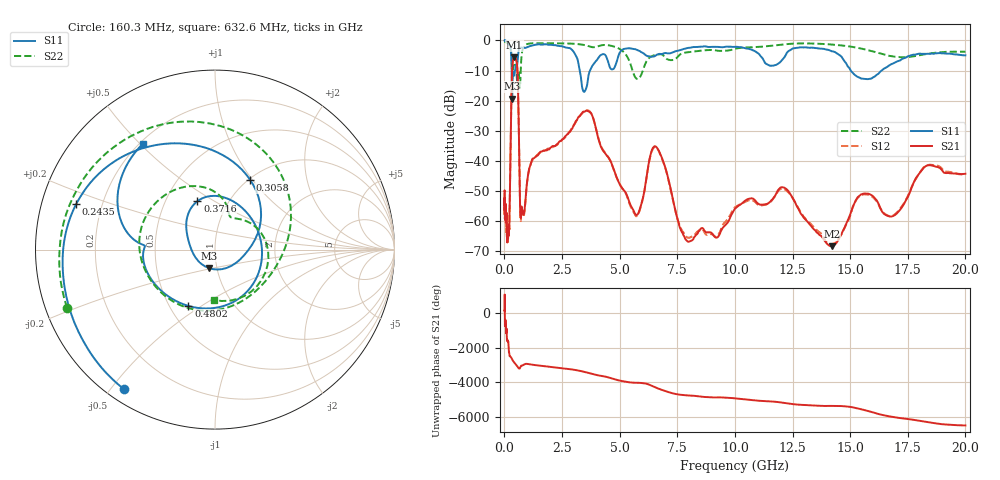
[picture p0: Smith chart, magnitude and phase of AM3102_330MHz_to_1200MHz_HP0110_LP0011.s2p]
! Date/Time: Tue, Sep 11, 2018 5:14 PM
! Network Analyzer: Agilent Technologies E8362B Rev: A.07.50.63
! Sweep from 0.010 to 20.000 GHz, 1601 Points, Sweep Type: LOG
! Power Supply: 4.949 V, 0.001 A
# Hz S DB R 50
!freq MagS11 AngS11 MagS21 AngS21 MagS12 AngS12 MagS22 AngS22
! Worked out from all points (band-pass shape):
!   1601 points, 10 MHz to 20 GHz, reference 50 ohm
!   highest |S21| = -5.58 dB at 426.5 MHz (marker M1); lowest = -68.3 dB at 14.21 GHz (marker M2)
!   |S21| within 3 dB of the highest: 343.4 MHz to 555.1 MHz (211.7 MHz wide, 47.1 % of centre)
!   lowest |S11| = -19.3 dB at 337.9 MHz (marker M3), VSWR 1.24, Z = 45.7 - j9.53 ohm
!   |S11| at or under -10 dB: 315 MHz to 461.3 MHz (146.3 MHz wide, 37.7 % of centre); 3.274 GHz to 3.714 GHz (440.5 MHz wide, 12.6 % of centre); 15.03 GHz to 16.37 GHz (1.34 GHz wide, 8.54 % of centre)
!   |S22| runs from -15.8 to -0.2 dB; largest |S21 - S12| = 0.0081
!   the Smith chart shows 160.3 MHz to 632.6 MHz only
!   S11 on the Smith chart (normalised r, x): 160.3 MHz: 0.05, -0.54; 243.5 MHz: 0.11, +0.16; 305.8 MHz: 1.02, +0.97; 371.6 MHz: 0.72, +0.42; 480.2 MHz: 0.62, -0.44; 632.6 MHz: 0.21, +0.51
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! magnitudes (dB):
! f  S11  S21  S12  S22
! 10 MHz  0.0  -50.1  -50.7  -0.2
! 35.55 MHz  0.0  -57.7  -56.3  -0.4
! 126.4 MHz  -0.4  -65.0  -62.6  -0.9
! 160.3 MHz  -0.6  -65.8  -64.9  -1.1
! 243.5 MHz  -1.8  -48.7  -48.7  -1.9
! 305.8 MHz  -7.2  -18.7  -18.7  -4.6
! 337.9 MHz  -19.3  -9.4  -9.4  -8.6
! 371.6 MHz  -10.8  -6.6  -6.7  -9.6
! 426.5 MHz  -11.6  -5.6  -5.6  -7.8
! 447.2 MHz  -10.7  -5.6  -5.7  -7.4
! 480.2 MHz  -9.2  -5.8  -5.9  -7.6
! 567.1 MHz  -7.4  -10.2  -10.3  -13.8
! 632.6 MHz  -2.9  -32.1  -32.2  -11.1
! 709 MHz  -2.4  -59.0  -60.0  -10.1
! 1.59 GHz  -1.4  -36.9  -37.0  -0.9
! 3.651 GHz  -11.6  -23.6  -23.3  -1.9
! 5.652 GHz  -2.9  -57.3  -57.7  -11.9
! 6.58 GHz  -4.9  -35.3  -35.5  -4.8
! 7.92 GHz  -2.5  -66.6  -65.4  -4.0
! 12.09 GHz  -6.1  -48.8  -49.2  -1.3
! 14.21 GHz  -3.6  -68.3  -67.6  -1.4
! 20 GHz  -4.9  -44.3  -44.7  -3.7
